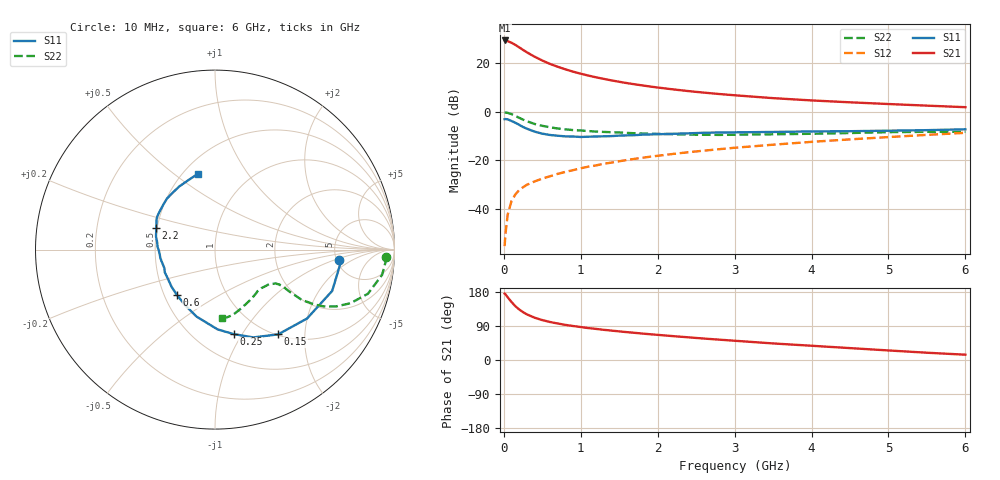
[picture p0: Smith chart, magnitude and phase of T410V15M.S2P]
! Infineon Technologies  Discrete & RF Semiconductors
! BFR182T
! Si NPN RF Bipolar Junction Transistor in SC75
! VCE = 10 V  IC = 15 mA
! Common Emitter S-Parameters:  October  1999
# GHz  S  MA  R  50
!  f  S11  S21  S12  S22
! GHz  MAG  ANG  MAG  ANG  MAG  ANG  MAG  ANG
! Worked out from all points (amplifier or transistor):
!   36 points, 10 MHz to 6 GHz, reference 50 ohm
!   highest |S21| = 29.3 dB at 10 MHz (marker M1)
!   |S21| within 3 dB of that: start of sweep to 207.3 MHz
!   unconditionally stable (mu >= 1): 933 MHz to 3.981 GHz
!   at 250 MHz: K = 0.52, MSG = 28.3 dB, |S12| = -31.1 dB
!   at 1.4 GHz: K = 1.07, MAG = 15.3 dB, |S12| = -21.0 dB
!   at 6 GHz: K = 0.88, MSG = 5.3 dB, |S12| = -8.7 dB
!   S11 on the Smith chart (normalised r, x): 10 MHz: 5.31, -1.15; 150 MHz: 1.02, -1.47; 250 MHz: 0.75, -0.92; 600 MHz: 0.58, -0.33; 2.2 GHz: 0.49, +0.14; 6 GHz: 0.59, +0.61
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0.01  0.6956 -4.6  29.1 175.2  0.0017 69.2  0.9558 -2.4
0.02  0.7031 -6.3  28.76 173.7  0.0029 85.0  0.9554 -3.4
0.05  0.6923 -19.4  28.18 165.4  0.0076 81.5  0.9416 -8.6
0.1  0.6407 -36.8  26.08 153.0  0.0145 75.9  0.8868 -16.1
0.15  0.589 -53.3  23.54 141.9  0.0198 68.6  0.8118 -21.6
0.2  0.5339 -66.4  20.96 133.3  0.0243 66.1  0.7442 -25.2
0.25  0.4819 -77.6  18.58 126.2  0.0278 62.2  0.6821 -27.6
0.3  0.4445 -88.2  16.57 120.4  0.0312 61.9  0.6333 -28.9
0.4  0.3871 -105.4  13.46 111.6  0.0366 61.3  0.5565 -30.1
0.5  0.3512 -118.6  11.24 105.3  0.0418 61.9  0.5094 -29.7
0.6  0.33 -129.9  9.58 100.3  0.0467 63.2  0.4749 -29.4
0.8  0.3088 -147.9  7.411 92.7  0.0574 64.5  0.4315 -28.7
0.9  0.3072 -155.4  6.63 89.7  0.0623 65.5  0.4164 -28.6
1.1  0.3042 -166.9  5.503 84.2  0.0737 66.2  0.3972 -28.9
1.3  0.31 -176.1  4.707 79.6  0.0847 66.9  0.3815 -29.7
1.6  0.324 173.5  3.858 73.5  0.101 67.2  0.3639 -31.5
2.2  0.3495 159.8  2.864 63.0  0.1345 66.8  0.3425 -37.4
2.8  0.3712 149.6  2.299 53.7  0.1683 65.0  0.3313 -44.5
3.5  0.3812 139.4  1.891 43.7  0.2083 62.4  0.3414 -53.7
4.5  0.3948 126.9  1.552 31.4  0.2681 57.6  0.3621 -68.0
5.5  0.4148 110.7  1.326 19.2  0.3318 52.3  0.3832 -79.9
6  0.432 103.0  1.232 14.0  0.3657 48.8  0.3841 -84.5
